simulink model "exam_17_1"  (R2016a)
settings: Solver=ode23tb  StartTime=0.0  StopTime=0.2  RelTol=1e-3
libraries: powerlib x9

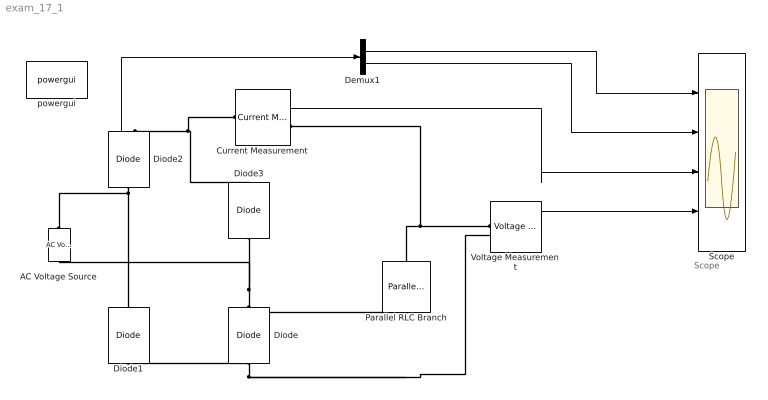
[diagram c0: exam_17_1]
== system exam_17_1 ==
  note: Scope
  AC Voltage Source : powerlib/Electrical Sources/AC Voltage Source  Amplitude=100  Phase=0  Frequency=50  SampleTime=0  Measurements=None  BusType=swing  Pref=10e3  Qref=0  Qmin=-inf  Qmax=+inf
  Current Measurement : powerlib/Measurements/Current Measurement  PhasorSimulation=off  OutputType=Complex  PSBequivalent=0
  Demux1 : Demux  Outputs=2
  Diode : powerlib/Power Electronics/Diode  Ron=0.001  Lon=0  Vf=0.8  IC=0  UseSnubber=off  Rs=500  Cs=250e-9  Measurements=off
  Diode1 : powerlib/Power Electronics/Diode  Ron=0.001  Lon=0  Vf=0.8  IC=0  UseSnubber=off  Rs=500  Cs=250e-9  Measurements=off
  Diode2 : powerlib/Power Electronics/Diode  Ron=0.001  Lon=0  Vf=0.8  IC=0  UseSnubber=off  Rs=500  Cs=250e-9  Measurements=on
  Diode3 : powerlib/Power Electronics/Diode  Ron=0.001  Lon=0  Vf=0.8  IC=0  UseSnubber=off  Rs=500  Cs=250e-9  Measurements=off
  Parallel RLC Branch : powerlib/Elements/Parallel RLC Branch  LConnTagsString=a  RConnTagsString=__new0  BranchType=R  Resistance=1  Inductance=1e-3  SetiL0=off  InitialCurrent=0  Capacitance=1e-6  Setx0=off  InitialVoltage=0  Measurements=None
  Scope : Scope  NumInputPorts=4
  Voltage Measurement : powerlib/Measurements/Voltage Measurement  PhasorSimulation=off  OutputType=Complex  PSBequivalent=0
  powergui : powerlib/powergui  Priority=1  SimulationMode=Continuous  SolverType=Tustin/Backward Euler (TBE)  SampleTime=50e-6  frequency=60  SPID=off  DisableSnubberDevices=off  DisableRonSwitches=off  DisableVfSwitches=off  SwTol=0  DisplayEquations=off  Interpol=off  ExternalGateDelay=off  methode=off  Ts=10  FunctionMessages=off  echomessages=off  HookPort=off  EnableUseOfTLC=off  x0status=blocks  frequencyindice=50  Pbase=100e6  ErrMax=1e-4  Iterations=50  UnitsV=kV  UnitsW=MW  buscounter=0  RestoreLinks=warning  ResistiveCurrentMeasurement=off  Frange=[0:2:500]  Ylog=off  Xlog=on  ShowGrid=off  save=off  variable=ZData  structure=0  ZoomFFT=off  StartTime=0.0  cycles=1  DisplayStyle=1  fundamental=60  FreqAxis=off  MaxFrequency=1000  frequencyindicesteady=1  RmsSteady=1  display=off
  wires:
  Demux1/1 -> Scope/1
  Demux1/2 -> Scope/2
  Current Measurement/1 -> Scope/3
  Voltage Measurement/1 -> Scope/4
  Diode2/1 -> Demux1/1
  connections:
  Diode2/LConn1 -- Diode1/RConn1 -- AC Voltage Source/RConn1
  Diode2/RConn1 -- Diode3/RConn1 -- Current Measurement/LConn1
  Diode/RConn1 -- AC Voltage Source/LConn1 -- Diode3/LConn1
  Voltage Measurement/LConn1 -- Parallel RLC Branch/LConn1 -- Current Measurement/RConn1
  Diode1/LConn1 -- Voltage Measurement/LConn2 -- Parallel RLC Branch/RConn1 -- Diode/LConn1
